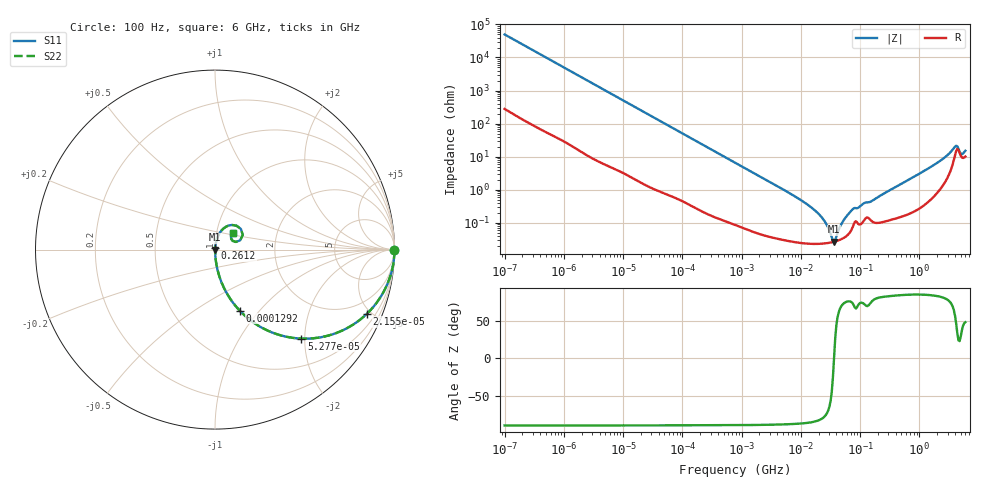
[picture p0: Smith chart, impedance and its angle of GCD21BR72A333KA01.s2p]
!Murata Part Number: GCD21BR72A333KA01
!These Parameters are Measured in Series Mode Connection
!Data Generated on Jan 08, 2026
!  o--ll--o
!Port1  Port2
!  o------o
!Operation Temp=25[degC], DC Bias Voltage=0[V]
!Freq. Start=100[Hz] Stop=6[GHz] 401[Steps]
# Hz S RI R 50
!Freq.(Hz) S11(Real) S11(Imag) S21(Real) S21(Imag) S12(Real) S12(Imag) S22(Real) S22(Imag)
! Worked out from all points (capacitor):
!   401 points, 100 Hz to 6 GHz, reference 50 ohm
!   read as one part in series: C = 32 nF near 109 Hz
!   lowest |Z| = 26.7 mohm at 36.42 MHz (marker M1)
!   series resonance near 36.34 MHz, so ESL is about 600 pH
!   S11 on the Smith chart (normalised r, x): 100 Hz: open; 21.55 kHz: 1.03, -4.70; 52.77 kHz: 1.01, -1.93; 129.2 kHz: 1.01, -0.79; 261.2 MHz: 1.00, +0.02; 6 GHz: 1.20, +0.22
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100  1 -0.00201  1.53e-05 0.00201  1.53e-05 0.00201  1 -0.00201
2008  0.9982 -0.0399  0.00181 0.0399  0.00181 0.0399  0.9982 -0.0399
7358  0.9783 -0.1426  0.0217 0.1426  0.0217 0.1426  0.9783 -0.1426
21550  0.8452 -0.3585  0.1548 0.3585  0.1548 0.3585  0.8452 -0.3585
40335  0.6123 -0.4837  0.3877 0.4837  0.3877 0.4837  0.6123 -0.4837
52766  0.4815 -0.4958  0.5185 0.4958  0.5185 0.4958  0.4815 -0.4958
129199  0.1375 -0.3399  0.8625 0.3399  0.8625 0.3399  0.1375 -0.3399
252896  0.0412 -0.194  0.9588 0.194  0.9588 0.194  0.0412 -0.194
774597  0.00527 -0.0662  0.9947 0.0662  0.9947 0.0662  0.00527 -0.0662
6644369  0.000331 -0.00762  0.9997 0.00762  0.9997 0.00762  0.000331 -0.00762
1.555665e7  0.000237 -0.00277  0.9998 0.00277  0.9998 0.00277  0.000237 -0.00277
2.434276e7  0.000237 -0.0012  0.9998 0.0012  0.9998 0.0012  0.000237 -0.0012
3.330331e7  0.000257 -0.000255  0.9997 0.000255  0.9997 0.000255  0.000257 -0.000255
3.64232e7  0.000266 6.6e-06  0.9997 -6.6e-06  0.9997 -6.6e-06  0.000266 6.6e-06
5.211241e7  0.000343 0.00109  0.9997 -0.00109  0.9997 -0.00109  0.000343 0.00109
7.455971e7  0.000721 0.00242  0.9993 -0.00242  0.9993 -0.00242  0.000721 0.00242
2.61201e8  0.00115 0.00784  0.9989 -0.00784  0.9989 -0.00784  0.00115 0.00784
3.124326e8  0.00127 0.00941  0.9987 -0.00941  0.9987 -0.00941  0.00127 0.00941
1.873145e9  0.0104 0.0585  0.9896 -0.0585  0.9896 -0.0585  0.0104 0.0585
4.009986e9  0.1193 0.1334  0.8807 -0.1334  0.8807 -0.1334  0.1193 0.1334
5.245841e9  0.0903 0.06  0.9097 -0.06  0.9097 -0.06  0.0903 0.06
6e9  0.101 0.0918  0.899 -0.0918  0.899 -0.0918  0.101 0.0918
